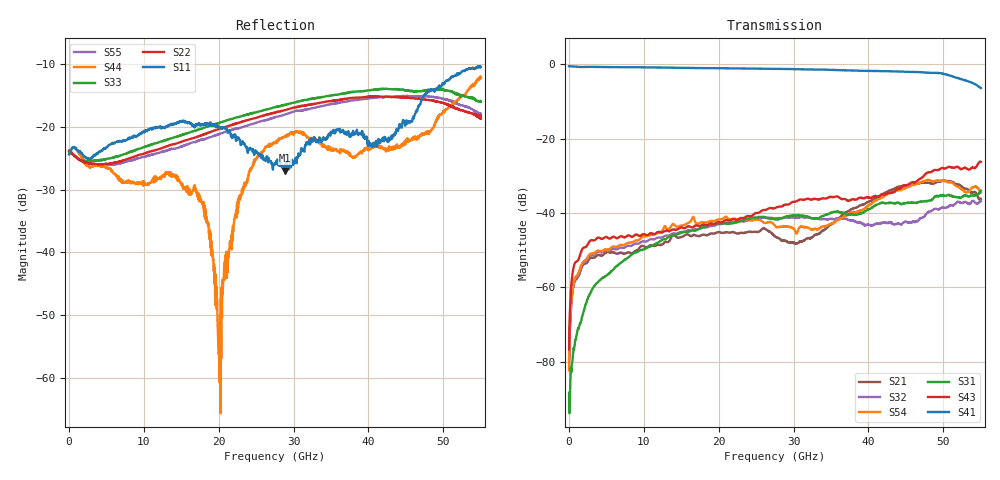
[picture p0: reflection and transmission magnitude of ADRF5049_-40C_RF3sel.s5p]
! Device  : ADRF5049
! Description: Silicon SP4T Switch Non-Reflective
! Frequency:  9kHz -  45 GHz
! Ports:
!  RFC = Port 1
!  RF1 = Port 2
!  RF2 = Port 3
!	 RF3 = Port 4
!  RF4 = Port 5
! VSS  =  +3.30 Volts
! VDD  =  -3.30 Volts
! EN  =  0.00 Volts
! LS  =  0.00 Volts
! V1  =  0.00 Volts
! V2  =  3.30 Volts
! Data:  Data was collected using an calibrated 4 port network analyzer.
! Notes: Analog Devices supplies this data as a sample of measured data
!  for this product.  Your particular data for this product may vary.
!  Data was taken at -40 degrees C.
!  Analog Devices reserves the right to change this data at anytime.
# hz S db R 50
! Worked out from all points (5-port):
!   1100 points, 50 MHz to 55 GHz, reference 50 ohm
!   strongest paths, dB at 50 MHz, 13.8 GHz, 27.55 GHz, 41.3 GHz, 55 GHz:
!     S41: -0.6, -1.0, -1.3, -1.9, -6.4
!     S43: -76.6, -44.5, -38.7, -35.5, -26.3
!     S31: -88.3, -46.1, -41.7, -37.6, -34.0
!     S54: -82.2, -43.1, -43.5, -36.3, -34.5
!     S32: -80.0, -45.6, -41.4, -42.9, -36.8
!     S21: -79.3, -46.1, -46.3, -35.8, -36.2
!   lowest |S11| = -27.0 dB at 28.85 GHz (marker M1), VSWR 1.09, Z = 49.1 - j4.33 ohm
!   |S11| at or under -10 dB: start of sweep to end of sweep
